(* Logix 5000 Program export KEP; software revision 30.00; part 9 of 15 *)

ADD_ON_INSTRUCTION B256_DINTtoE   (* revision 1.0 20170916, vendor Kenneth A. Fischer *)
// Convert 256-bit value using 8 32-bit pieces into 256-bit value using 32 8-bit pieces
// Revision note:
// Rev1.0: 20170916 - Initial Release
VAR_IN_OUT
   Inp_DINT : DINT[8]; {required}
   Out_E : DINT[32]; {required}
END_VAR
VAR
   i : INT;
   j : INT;
   D_SHR : D_SHR;
   TEMP : DINT;
END_VAR

ROUTINE Logic   (* ladder *)
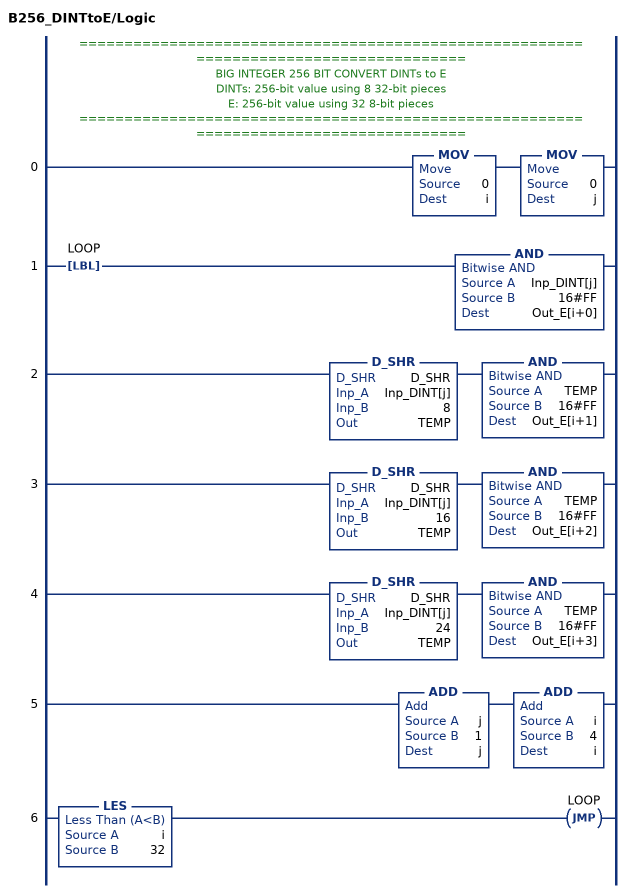
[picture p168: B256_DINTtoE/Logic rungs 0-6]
   // ======================================================================================
   // BIG INTEGER 256 BIT CONVERT DINTs to E
   // DINTs: 256-bit value using 8 32-bit pieces
   // E: 256-bit value using 32 8-bit pieces
   // ======================================================================================
   0: MOV(0,i)MOV(0,j);
   1: LBL(LOOP)AND(Inp_DINT[j],16#FF,Out_E[i+0]);
   2: D_SHR(D_SHR,Inp_DINT[j],8,TEMP)AND(TEMP,16#FF,Out_E[i+1]);
   3: D_SHR(D_SHR,Inp_DINT[j],16,TEMP)AND(TEMP,16#FF,Out_E[i+2]);
   4: D_SHR(D_SHR,Inp_DINT[j],24,TEMP)AND(TEMP,16#FF,Out_E[i+3]);
   5: ADD(j,1,j)ADD(i,4,i);
   6: LES(i,32)JMP(LOOP);
END_ROUTINE
END_ADD_ON_INSTRUCTION

ADD_ON_INSTRUCTION B256_EtoDINT   (* revision 1.0 20170916, vendor Kenneth A. Fischer *)
// Convert 256-bit value using 32 8-bit pieces into 256-bit value using 8 32-bit pieces
// Revision note:
// Rev1.0: 20170916 - Initial Release
VAR_IN_OUT
   Inp_E : DINT[32]; {required}
   Out_DINT : DINT[8]; {required}
END_VAR
VAR
   D_SHL : D_SHL;
   i : INT;
   j : INT;
   TEMP : DINT;
END_VAR

ROUTINE Logic   (* ladder *)
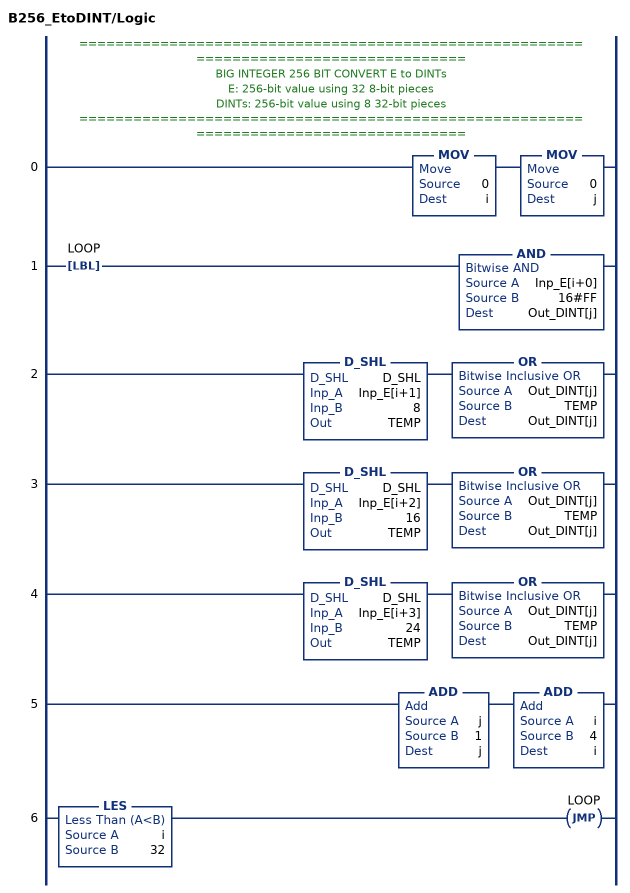
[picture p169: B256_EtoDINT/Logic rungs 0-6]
   // ======================================================================================
   // BIG INTEGER 256 BIT CONVERT E to DINTs
   // E: 256-bit value using 32 8-bit pieces
   // DINTs: 256-bit value using 8 32-bit pieces
   // ======================================================================================
   0: MOV(0,i)MOV(0,j);
   1: LBL(LOOP)AND(Inp_E[i+0],16#FF,Out_DINT[j]);
   2: D_SHL(D_SHL,Inp_E[i+1],8,TEMP)OR(Out_DINT[j],TEMP,Out_DINT[j]);
   3: D_SHL(D_SHL,Inp_E[i+2],16,TEMP)OR(Out_DINT[j],TEMP,Out_DINT[j]);
   4: D_SHL(D_SHL,Inp_E[i+3],24,TEMP)OR(Out_DINT[j],TEMP,Out_DINT[j]);
   5: ADD(j,1,j)ADD(i,4,i);
   6: LES(i,32)JMP(LOOP);
END_ROUTINE
END_ADD_ON_INSTRUCTION

ADD_ON_INSTRUCTION D_ROTR   (* revision 1.0 20170524, vendor Kenneth A. Fischer *)
// DINT circular right shift (rotation) of the 32-bit argument Inp_A by Inp_B bits
// Revision note:
// Rev1.0: 20170524 - Initial Release
VAR_IN_OUT
   Inp_A : DINT; {required}   // 64-bit Integer to be right circular rotated
END_VAR
VAR_INPUT
   Inp_B : INT; {required}   // Number of Inp_A bit rotations
END_VAR
VAR_IN_OUT
   Out : DINT; {required}   // Result
END_VAR
VAR
   Wrk_InpA : DINT[2];
   BSR_Cntrl : CONTROL := (LEN := 32);
   Source_Bit : BOOL;
   ONS : BOOL;
END_VAR

ROUTINE Logic   (* ladder *)
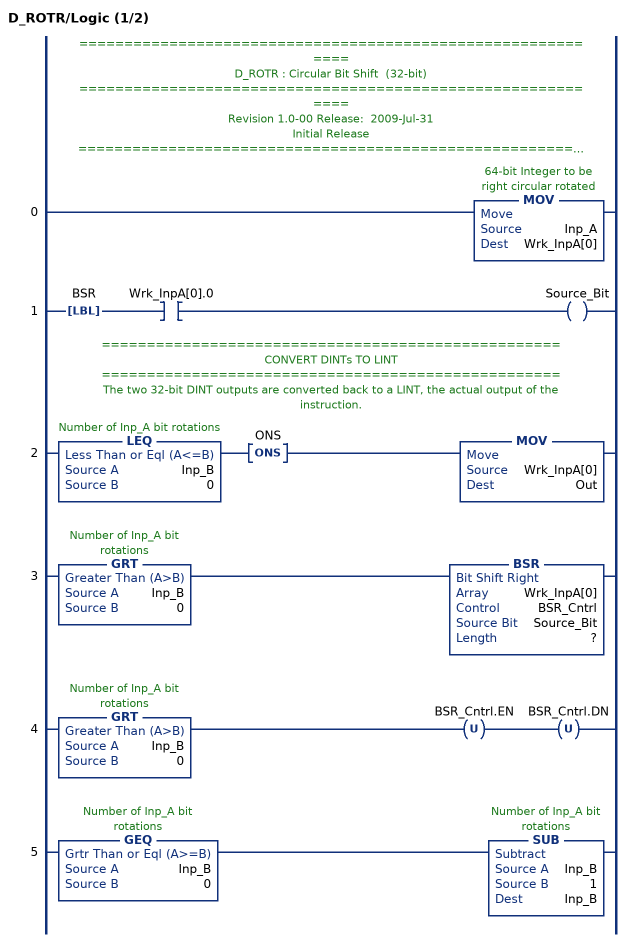
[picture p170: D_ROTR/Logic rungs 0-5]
   // ============================================================
   // D_ROTR : Circular Bit Shift  (32-bit)
   // ============================================================
   // Revision 1.0-00 Release:  2009-Jul-31
   // Initial Release
   // ============================================================
   // Performs a circular right shift rotation of the 32-bit argument Inp_A by the
   // number of bits defined in the 16-bit argument Inp_B.
   0: MOV(Inp_A,Wrk_InpA[0]);
   1: LBL(BSR)XIC(Wrk_InpA[0].0)OTE(Source_Bit);
   // ===================================================
   // CONVERT DINTs TO LINT
   // ===================================================
   // The two 32-bit DINT outputs are converted back to a LINT, the actual output of the instruction.
   2: LEQ(Inp_B,0)ONS(ONS)MOV(Wrk_InpA[0],Out);
   3: GRT(Inp_B,0)BSR(Wrk_InpA[0],BSR_Cntrl,Source_Bit,?);
   4: GRT(Inp_B,0)OTU(BSR_Cntrl.EN)OTU(BSR_Cntrl.DN);
   5: GEQ(Inp_B,0)SUB(Inp_B,1,Inp_B);
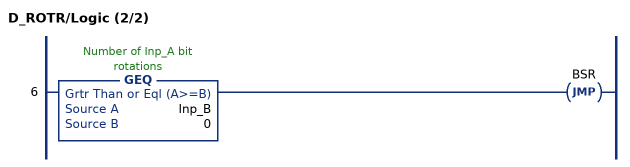
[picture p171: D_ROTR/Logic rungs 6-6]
   6: GEQ(Inp_B,0)JMP(BSR);
END_ROUTINE
END_ADD_ON_INSTRUCTION

ADD_ON_INSTRUCTION VMAC   (* revision 1.0 20170524, vendor Kenneth A. Fischer *)
// Variable Round MAC
// Revision note:
// Rev1.0: 20170524 - Initial Release
VAR_IN_OUT
   Inp_KEY : DINT[8]; {required}
   Inp_MSG : DINT[500]; {required}
END_VAR
VAR_INPUT
   Inp_LEN : DINT; {required}   // LENGTH INPUT OF MSG IN NUMBER OF DINTS
   Inp_ROUNDS : DINT; {required}
END_VAR
VAR_IN_OUT
   Out_VMAC : DINT[8]; {required}
        [0]   // HashBuffer_A
        [1]   // HashBuffer_B
        [2]   // HashBuffer_C
        [3]   // HashBuffer_D
        [4]   // HashBuffer_E
        [5]   // HashBuffer_F
        [6]   // HashBuffer_G
        [7]   // HashBuffer_H
END_VAR
VAR
   MajFunc : DINT;
   HashBuffer_H : DINT;
   HashBuffer_G : DINT;
   HashBuffer_F : DINT;
   HashBuffer_E : DINT;
   HashBuffer_D : DINT;
   HashBuffer_C : DINT;
   HashBuffer_B : DINT;
   HashBuffer_A : DINT;
   W : DINT[64];   // MESSAGE SCHEDULE
   tmp : DINT[20];
   T2 : DINT;
   T1 : DINT;
   t : INT;
   M : INT;   // MESSAGE INCREMENTS
   SigmaE : DINT;
   SigmaA : DINT;
   Sigma1 : DINT;
   Sigma0 : DINT;
   i : INT;
   x : INT;
   HashBufferInput_H : DINT;
   HashBufferInput_G : DINT;
   HashBufferInput_F : DINT;
   HashBufferInput_E : DINT;
   HashBufferInput_D : DINT;
   HashBufferInput_C : DINT;
   HashBufferInput_B : DINT;
   HashBufferInput_A : DINT;
   CondFunc : DINT;
   K : DINT[64];
   LENGTH_BITS : DINT;   // LENGTH OF MSG IN BITS
   LENGTH_MODULO : DINT;
   NUM_PADDING_BITS : DINT;   // NUMBER OF BITS NEEDED FOR PADDING
   NUM_PADDING_DINTS : DINT;   // NUMBER OF DINTS NEEDED FOR PADDING
   PADDING_COUNTER : DINT;
   TOTAL_MSG_LENGTH_MINUS_16 : DINT;
   D_ROTR : D_ROTR;
   D_SHR : D_SHR;
   ROUNDS : DINT;
   n : INT;
   KeyIndex : DINT;
   RotationIndex : DINT;
   IndexedKey : DINT;
END_VAR

ROUTINE Logic   (* ladder *)
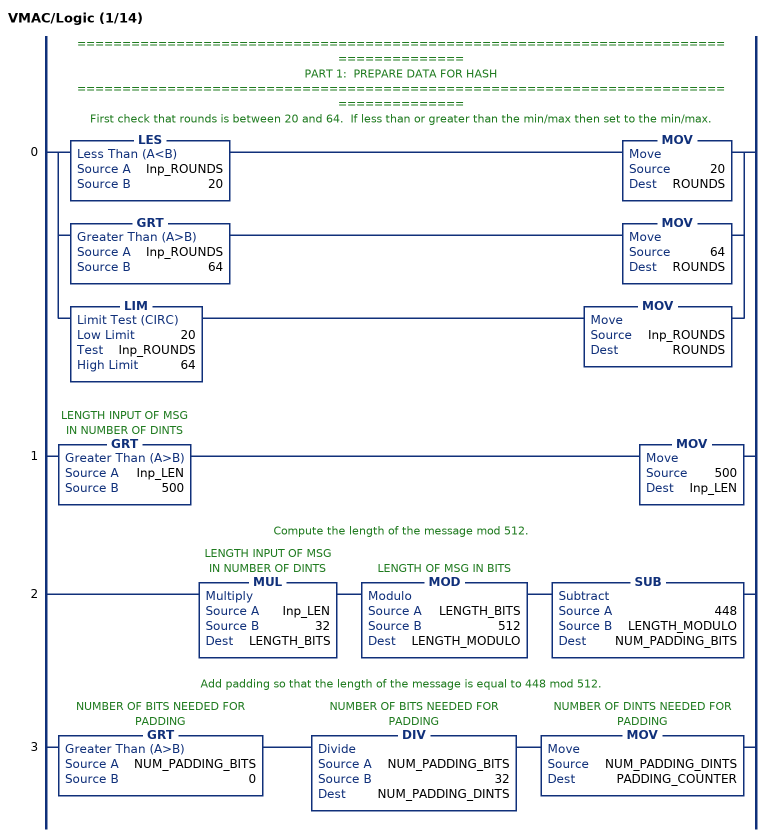
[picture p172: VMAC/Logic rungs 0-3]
   // ======================================================================================
   // PART 1:  PREPARE DATA FOR HASH
   // ======================================================================================
   // First check that rounds is between 20 and 64.  If less than or greater than the min/max then set to the min/max.
   0: [LES(Inp_ROUNDS,20) MOV(20,ROUNDS) ,GRT(Inp_ROUNDS,64) MOV(64,ROUNDS) ,LIM(20,Inp_ROUNDS,64) MOV(Inp_ROUNDS,ROUNDS) ];
   1: GRT(Inp_LEN,500)MOV(500,Inp_LEN);
   // Compute the length of the message mod 512.
   2: MUL(Inp_LEN,32,LENGTH_BITS)MOD(LENGTH_BITS,512,LENGTH_MODULO)SUB(448,LENGTH_MODULO,NUM_PADDING_BITS);
   // Add padding so that the length of the message is equal to 448 mod 512.
   3: GRT(NUM_PADDING_BITS,0)DIV(NUM_PADDING_BITS,32,NUM_PADDING_DINTS)MOV(NUM_PADDING_DINTS,PADDING_COUNTER);
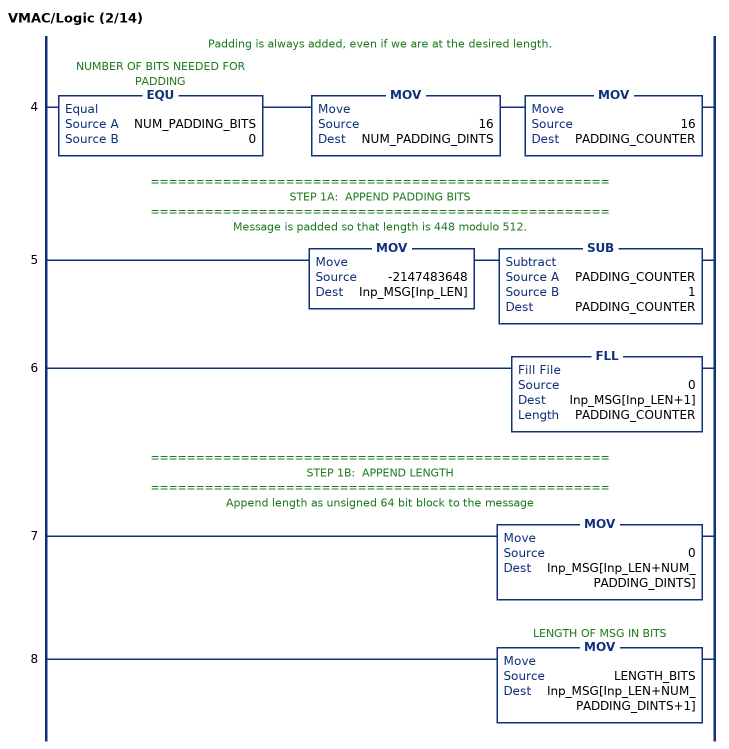
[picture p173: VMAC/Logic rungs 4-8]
   // Padding is always added, even if we are at the desired length.
   4: EQU(NUM_PADDING_BITS,0)MOV(16,NUM_PADDING_DINTS)MOV(16,PADDING_COUNTER);
   // ===================================================
   // STEP 1A:  APPEND PADDING BITS
   // ===================================================
   // Message is padded so that length is 448 modulo 512.
   5: MOV(-2147483648,Inp_MSG[Inp_LEN])SUB(PADDING_COUNTER,1,PADDING_COUNTER);
   6: FLL(0,Inp_MSG[Inp_LEN+1],PADDING_COUNTER);
   // ===================================================
   // STEP 1B:  APPEND LENGTH
   // ===================================================
   // Append length as unsigned 64 bit block to the message
   7: MOV(0,Inp_MSG[Inp_LEN+NUM_PADDING_DINTS]);
   8: MOV(LENGTH_BITS,Inp_MSG[Inp_LEN+NUM_PADDING_DINTS+1]);
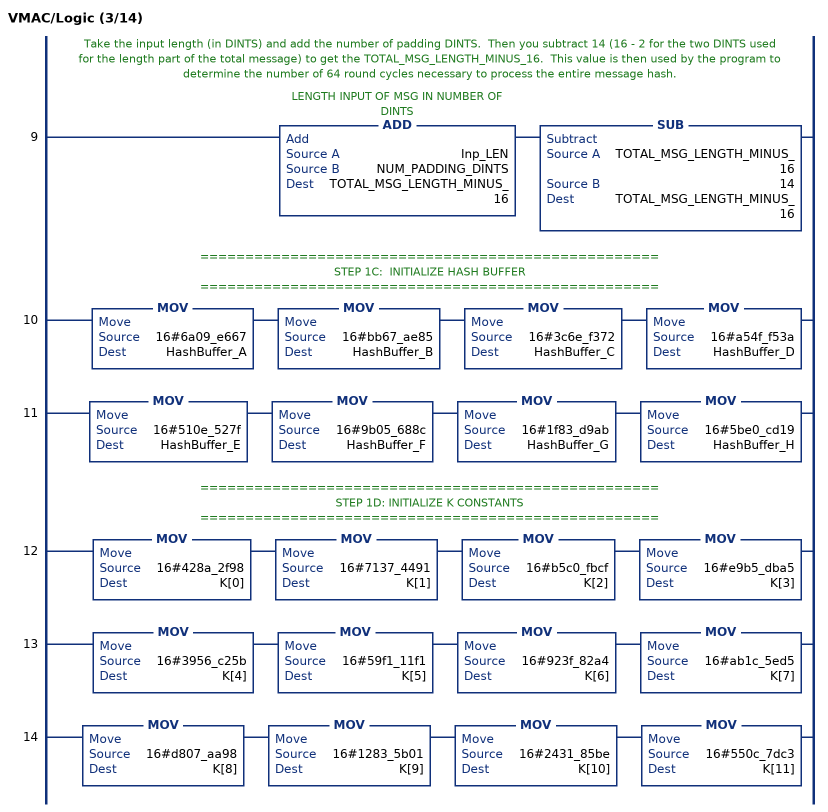
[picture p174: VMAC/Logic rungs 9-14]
   // Take the input length (in DINTS) and add the number of padding DINTS.  Then you subtract 14 (16 - 2 for the two DINTS used for the length part of the total message) to get the TOTAL_MSG_LENGTH_MINUS_16.  This value is then used by the program to determine the number of 64 round cycles necessary to process the entire message hash.
   9: ADD(Inp_LEN,NUM_PADDING_DINTS,TOTAL_MSG_LENGTH_MINUS_16)SUB(TOTAL_MSG_LENGTH_MINUS_16,14,TOTAL_MSG_LENGTH_MINUS_16);
   // ===================================================
   // STEP 1C:  INITIALIZE HASH BUFFER
   // ===================================================
   10: MOV(16#6a09_e667,HashBuffer_A)MOV(16#bb67_ae85,HashBuffer_B)MOV(16#3c6e_f372,HashBuffer_C)MOV(16#a54f_f53a,HashBuffer_D);
   11: MOV(16#510e_527f,HashBuffer_E)MOV(16#9b05_688c,HashBuffer_F)MOV(16#1f83_d9ab,HashBuffer_G)MOV(16#5be0_cd19,HashBuffer_H);
   // ===================================================
   // STEP 1D: INITIALIZE K CONSTANTS
   // ===================================================
   12: MOV(16#428a_2f98,K[0])MOV(16#7137_4491,K[1])MOV(16#b5c0_fbcf,K[2])MOV(16#e9b5_dba5,K[3]);
   13: MOV(16#3956_c25b,K[4])MOV(16#59f1_11f1,K[5])MOV(16#923f_82a4,K[6])MOV(16#ab1c_5ed5,K[7]);
   14: MOV(16#d807_aa98,K[8])MOV(16#1283_5b01,K[9])MOV(16#2431_85be,K[10])MOV(16#550c_7dc3,K[11]);
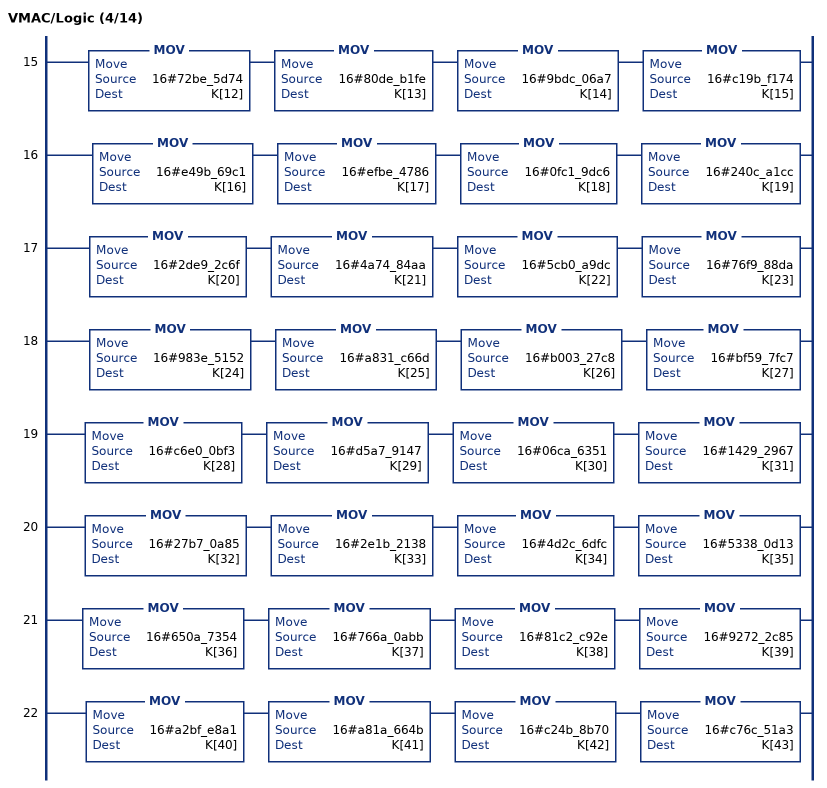
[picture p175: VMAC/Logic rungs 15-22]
   15: MOV(16#72be_5d74,K[12])MOV(16#80de_b1fe,K[13])MOV(16#9bdc_06a7,K[14])MOV(16#c19b_f174,K[15]);
   16: MOV(16#e49b_69c1,K[16])MOV(16#efbe_4786,K[17])MOV(16#0fc1_9dc6,K[18])MOV(16#240c_a1cc,K[19]);
   17: MOV(16#2de9_2c6f,K[20])MOV(16#4a74_84aa,K[21])MOV(16#5cb0_a9dc,K[22])MOV(16#76f9_88da,K[23]);
   18: MOV(16#983e_5152,K[24])MOV(16#a831_c66d,K[25])MOV(16#b003_27c8,K[26])MOV(16#bf59_7fc7,K[27]);
   19: MOV(16#c6e0_0bf3,K[28])MOV(16#d5a7_9147,K[29])MOV(16#06ca_6351,K[30])MOV(16#1429_2967,K[31]);
   20: MOV(16#27b7_0a85,K[32])MOV(16#2e1b_2138,K[33])MOV(16#4d2c_6dfc,K[34])MOV(16#5338_0d13,K[35]);
   21: MOV(16#650a_7354,K[36])MOV(16#766a_0abb,K[37])MOV(16#81c2_c92e,K[38])MOV(16#9272_2c85,K[39]);
   22: MOV(16#a2bf_e8a1,K[40])MOV(16#a81a_664b,K[41])MOV(16#c24b_8b70,K[42])MOV(16#c76c_51a3,K[43]);
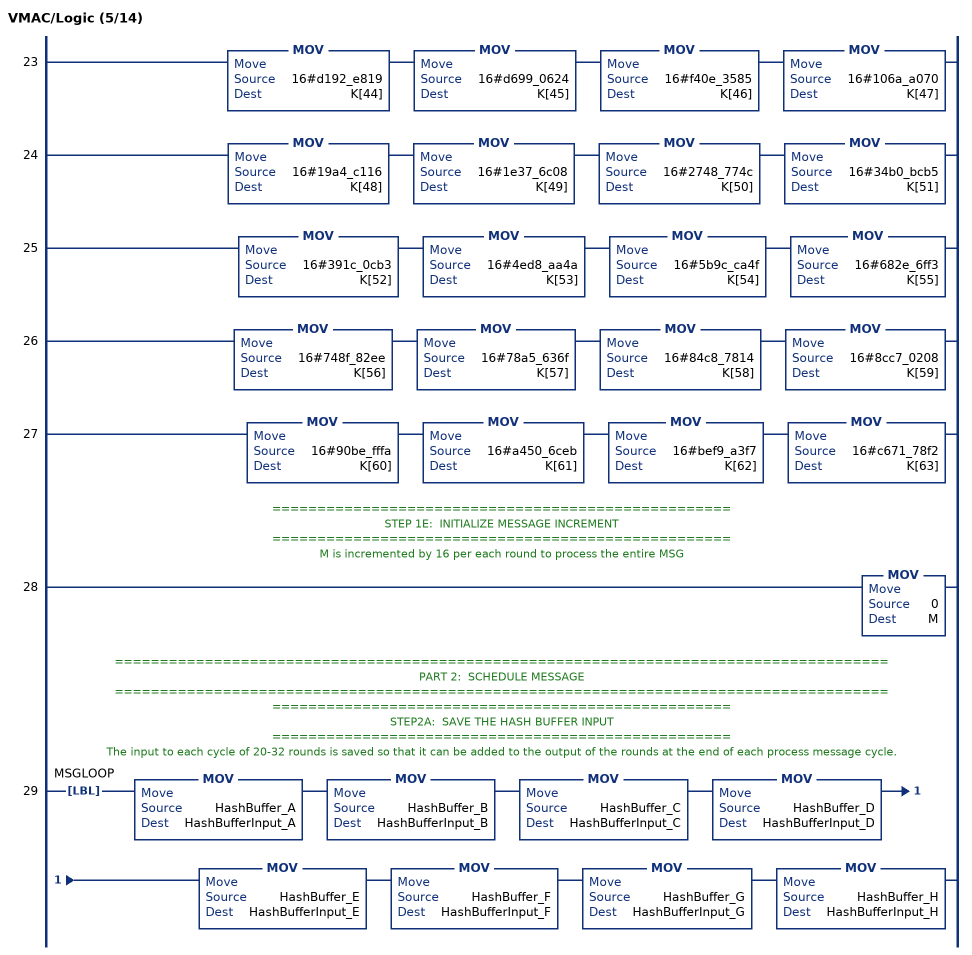
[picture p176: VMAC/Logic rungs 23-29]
   23: MOV(16#d192_e819,K[44])MOV(16#d699_0624,K[45])MOV(16#f40e_3585,K[46])MOV(16#106a_a070,K[47]);
   24: MOV(16#19a4_c116,K[48])MOV(16#1e37_6c08,K[49])MOV(16#2748_774c,K[50])MOV(16#34b0_bcb5,K[51]);
   25: MOV(16#391c_0cb3,K[52])MOV(16#4ed8_aa4a,K[53])MOV(16#5b9c_ca4f,K[54])MOV(16#682e_6ff3,K[55]);
   26: MOV(16#748f_82ee,K[56])MOV(16#78a5_636f,K[57])MOV(16#84c8_7814,K[58])MOV(16#8cc7_0208,K[59]);
   27: MOV(16#90be_fffa,K[60])MOV(16#a450_6ceb,K[61])MOV(16#bef9_a3f7,K[62])MOV(16#c671_78f2,K[63]);
   // ===================================================
   // STEP 1E:  INITIALIZE MESSAGE INCREMENT
   // ===================================================
   // M is incremented by 16 per each round to process the entire MSG
   28: MOV(0,M);
   // ======================================================================================
   // PART 2:  SCHEDULE MESSAGE
   // ======================================================================================
   // ===================================================
   // STEP2A:  SAVE THE HASH BUFFER INPUT
   // ===================================================
   // The input to each cycle of 20-32 rounds is saved so that it can be added to the output of the rounds at the end of each process message cycle.
   29: LBL(MSGLOOP)MOV(HashBuffer_A,HashBufferInput_A)MOV(HashBuffer_B,HashBufferInput_B)MOV(HashBuffer_C,HashBufferInput_C)MOV(HashBuffer_D,HashBufferInput_D)MOV(HashBuffer_E,HashBufferInput_E)MOV(HashBuffer_F,HashBufferInput_F)MOV(HashBuffer_G,HashBufferInput_G)MOV(HashBuffer_H,HashBufferInput_H);
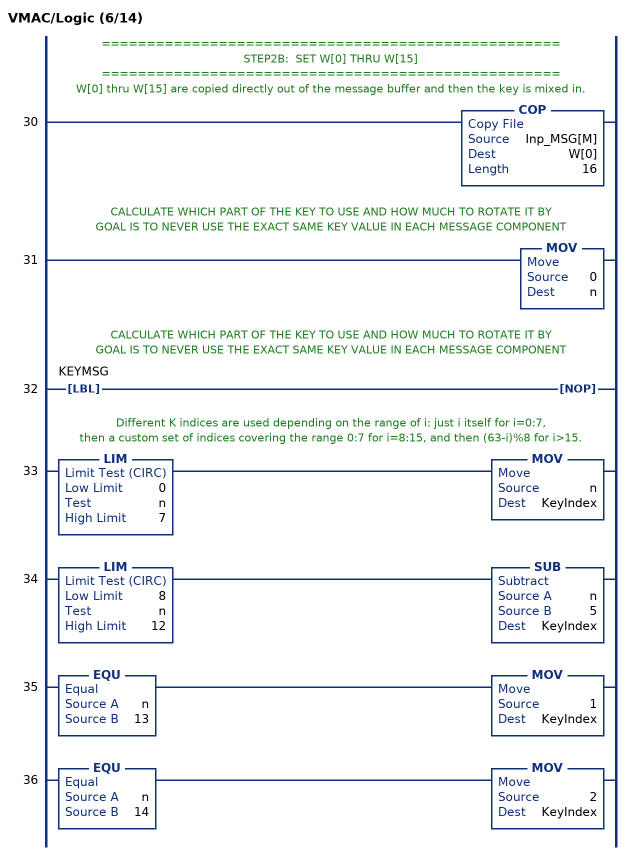
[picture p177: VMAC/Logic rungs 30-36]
   // ===================================================
   // STEP2B:  SET W[0] THRU W[15]
   // ===================================================
   // W[0] thru W[15] are copied directly out of the message buffer and then the key is mixed in.
   30: COP(Inp_MSG[M],W[0],16);
   // CALCULATE WHICH PART OF THE KEY TO USE AND HOW MUCH TO ROTATE IT BY
   // GOAL IS TO NEVER USE THE EXACT SAME KEY VALUE IN EACH MESSAGE COMPONENT
   31: MOV(0,n);
   // CALCULATE WHICH PART OF THE KEY TO USE AND HOW MUCH TO ROTATE IT BY
   // GOAL IS TO NEVER USE THE EXACT SAME KEY VALUE IN EACH MESSAGE COMPONENT
   32: LBL(KEYMSG)NOP();
   // Different K indices are used depending on the range of i: just i itself for i=0:7,
   // then a custom set of indices covering the range 0:7 for i=8:15, and then (63-i)%8 for i>15.
   33: LIM(0,n,7)MOV(n,KeyIndex);
   34: LIM(8,n,12)SUB(n,5,KeyIndex);
   35: EQU(n,13)MOV(1,KeyIndex);
   36: EQU(n,14)MOV(2,KeyIndex);
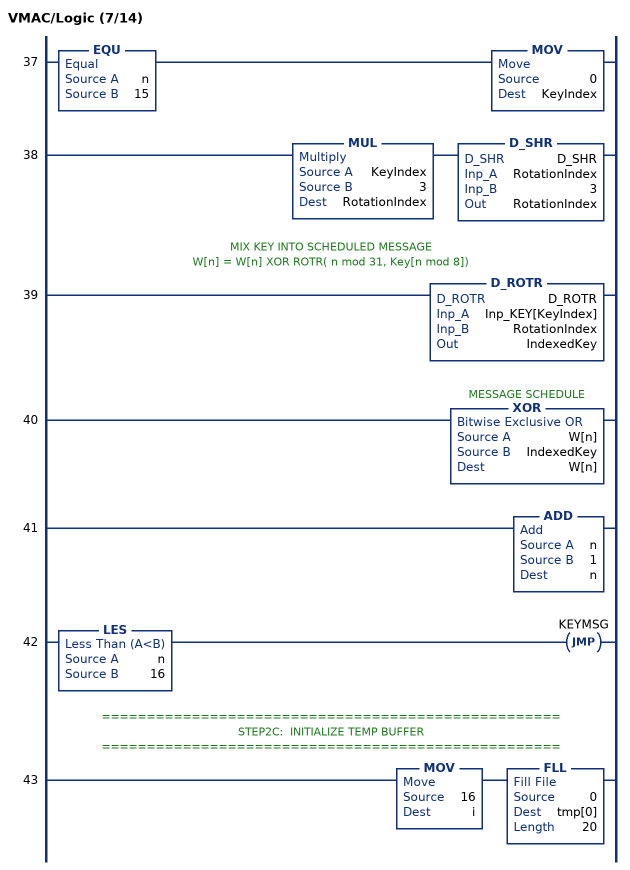
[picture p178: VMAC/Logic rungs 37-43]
   37: EQU(n,15)MOV(0,KeyIndex);
   38: MUL(KeyIndex,3,RotationIndex)D_SHR(D_SHR,RotationIndex,3,RotationIndex);
   // MIX KEY INTO SCHEDULED MESSAGE
   // W[n] = W[n] XOR ROTR( n mod 31, Key[n mod 8])
   39: D_ROTR(D_ROTR,Inp_KEY[KeyIndex],RotationIndex,IndexedKey);
   40: XOR(W[n],IndexedKey,W[n]);
   41: ADD(n,1,n);
   42: LES(n,16)JMP(KEYMSG);
   // ===================================================
   // STEP2C:  INITIALIZE TEMP BUFFER
   // ===================================================
   43: MOV(16,i)FLL(0,tmp[0],20);
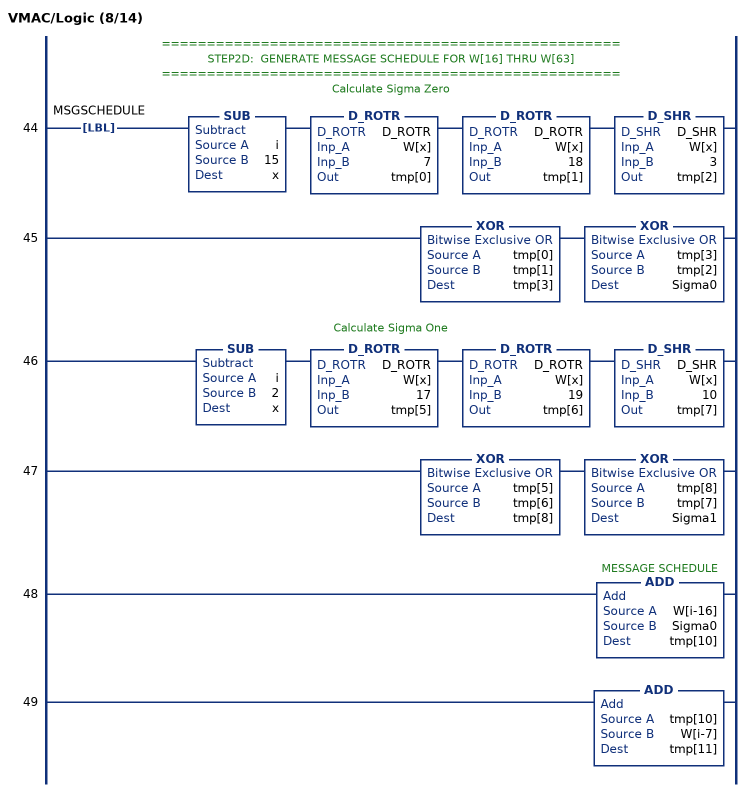
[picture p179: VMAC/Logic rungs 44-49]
   // ===================================================
   // STEP2D:  GENERATE MESSAGE SCHEDULE FOR W[16] THRU W[63]
   // ===================================================
   // Calculate Sigma Zero
   44: LBL(MSGSCHEDULE)SUB(i,15,x)D_ROTR(D_ROTR,W[x],7,tmp[0])D_ROTR(D_ROTR,W[x],18,tmp[1])D_SHR(D_SHR,W[x],3,tmp[2]);
   45: XOR(tmp[0],tmp[1],tmp[3])XOR(tmp[3],tmp[2],Sigma0);
   // Calculate Sigma One
   46: SUB(i,2,x)D_ROTR(D_ROTR,W[x],17,tmp[5])D_ROTR(D_ROTR,W[x],19,tmp[6])D_SHR(D_SHR,W[x],10,tmp[7]);
   47: XOR(tmp[5],tmp[6],tmp[8])XOR(tmp[8],tmp[7],Sigma1);
   48: ADD(W[i-16],Sigma0,tmp[10]);
   49: ADD(tmp[10],W[i-7],tmp[11]);
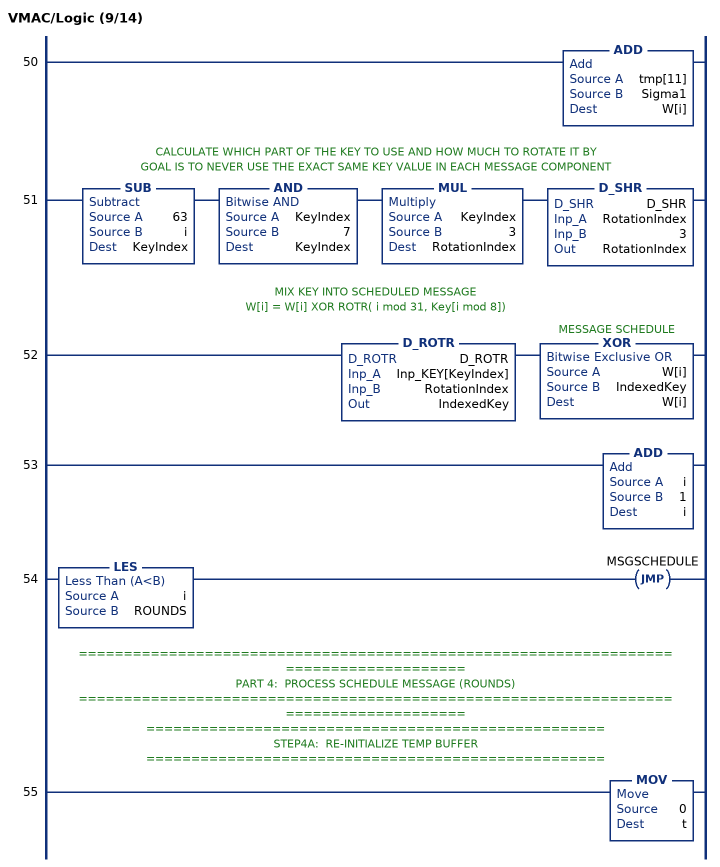
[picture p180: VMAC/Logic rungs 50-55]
   50: ADD(tmp[11],Sigma1,W[i]);
   // CALCULATE WHICH PART OF THE KEY TO USE AND HOW MUCH TO ROTATE IT BY
   // GOAL IS TO NEVER USE THE EXACT SAME KEY VALUE IN EACH MESSAGE COMPONENT
   51: SUB(63,i,KeyIndex)AND(KeyIndex,7,KeyIndex)MUL(KeyIndex,3,RotationIndex)D_SHR(D_SHR,RotationIndex,3,RotationIndex);
   // MIX KEY INTO SCHEDULED MESSAGE
   // W[i] = W[i] XOR ROTR( i mod 31, Key[i mod 8])
   52: D_ROTR(D_ROTR,Inp_KEY[KeyIndex],RotationIndex,IndexedKey)XOR(W[i],IndexedKey,W[i]);
   53: ADD(i,1,i);
   54: LES(i,ROUNDS)JMP(MSGSCHEDULE);
   // ======================================================================================
   // PART 4:  PROCESS SCHEDULE MESSAGE (ROUNDS)
   // ======================================================================================
   // ===================================================
   // STEP4A:  RE-INITIALIZE TEMP BUFFER
   // ===================================================
   55: MOV(0,t);
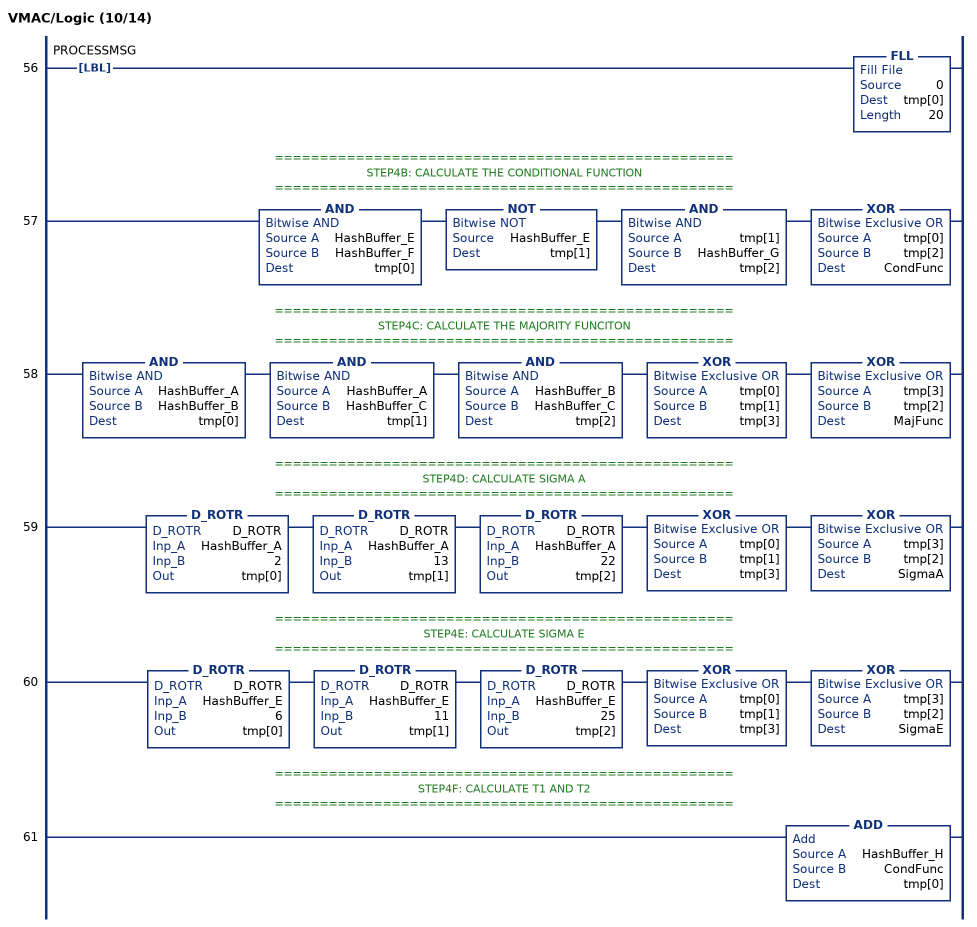
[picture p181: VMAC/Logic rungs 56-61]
   56: LBL(PROCESSMSG)FLL(0,tmp[0],20);
   // ===================================================
   // STEP4B: CALCULATE THE CONDITIONAL FUNCTION
   // ===================================================
   57: AND(HashBuffer_E,HashBuffer_F,tmp[0])NOT(HashBuffer_E,tmp[1])AND(tmp[1],HashBuffer_G,tmp[2])XOR(tmp[0],tmp[2],CondFunc);
   // ===================================================
   // STEP4C: CALCULATE THE MAJORITY FUNCITON
   // ===================================================
   58: AND(HashBuffer_A,HashBuffer_B,tmp[0])AND(HashBuffer_A,HashBuffer_C,tmp[1])AND(HashBuffer_B,HashBuffer_C,tmp[2])XOR(tmp[0],tmp[1],tmp[3])XOR(tmp[3],tmp[2],MajFunc);
   // ===================================================
   // STEP4D: CALCULATE SIGMA A
   // ===================================================
   59: D_ROTR(D_ROTR,HashBuffer_A,2,tmp[0])D_ROTR(D_ROTR,HashBuffer_A,13,tmp[1])D_ROTR(D_ROTR,HashBuffer_A,22,tmp[2])XOR(tmp[0],tmp[1],tmp[3])XOR(tmp[3],tmp[2],SigmaA);
   // ===================================================
   // STEP4E: CALCULATE SIGMA E
   // ===================================================
   60: D_ROTR(D_ROTR,HashBuffer_E,6,tmp[0])D_ROTR(D_ROTR,HashBuffer_E,11,tmp[1])D_ROTR(D_ROTR,HashBuffer_E,25,tmp[2])XOR(tmp[0],tmp[1],tmp[3])XOR(tmp[3],tmp[2],SigmaE);
   // ===================================================
   // STEP4F: CALCULATE T1 AND T2
   // ===================================================
   61: ADD(HashBuffer_H,CondFunc,tmp[0]);
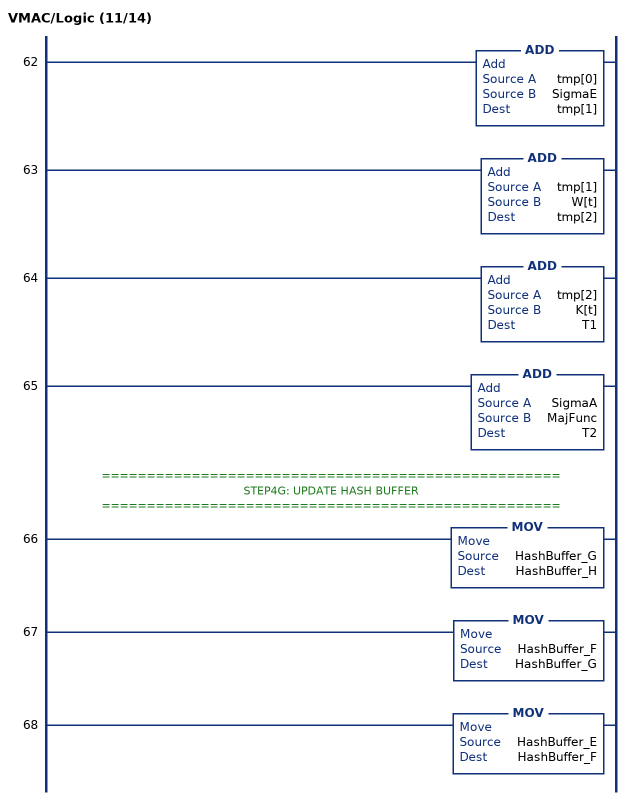
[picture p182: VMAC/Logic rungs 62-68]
   62: ADD(tmp[0],SigmaE,tmp[1]);
   63: ADD(tmp[1],W[t],tmp[2]);
   64: ADD(tmp[2],K[t],T1);
   65: ADD(SigmaA,MajFunc,T2);
   // ===================================================
   // STEP4G: UPDATE HASH BUFFER
   // ===================================================
   66: MOV(HashBuffer_G,HashBuffer_H);
   67: MOV(HashBuffer_F,HashBuffer_G);
   68: MOV(HashBuffer_E,HashBuffer_F);
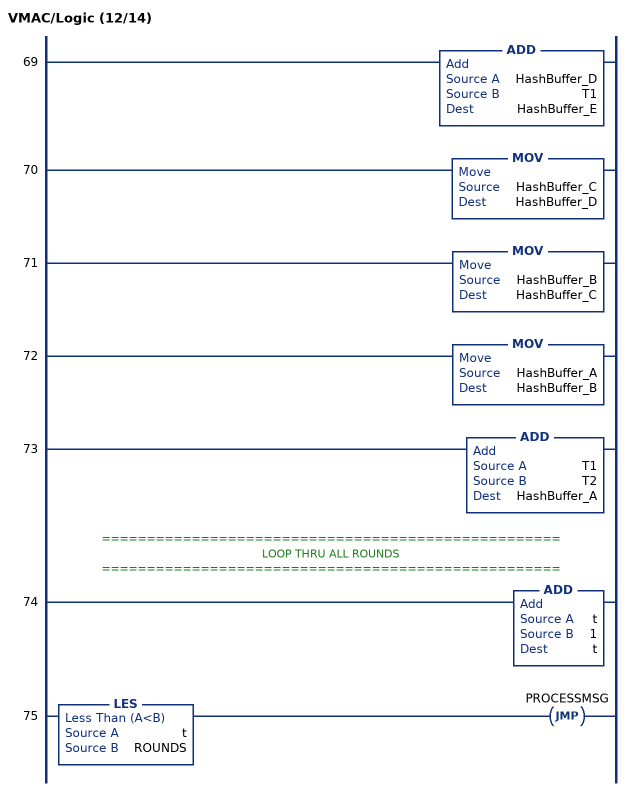
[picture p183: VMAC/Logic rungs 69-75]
   69: ADD(HashBuffer_D,T1,HashBuffer_E);
   70: MOV(HashBuffer_C,HashBuffer_D);
   71: MOV(HashBuffer_B,HashBuffer_C);
   72: MOV(HashBuffer_A,HashBuffer_B);
   73: ADD(T1,T2,HashBuffer_A);
   // ===================================================
   // LOOP THRU ALL ROUNDS
   // ===================================================
   74: ADD(t,1,t);
   75: LES(t,ROUNDS)JMP(PROCESSMSG);
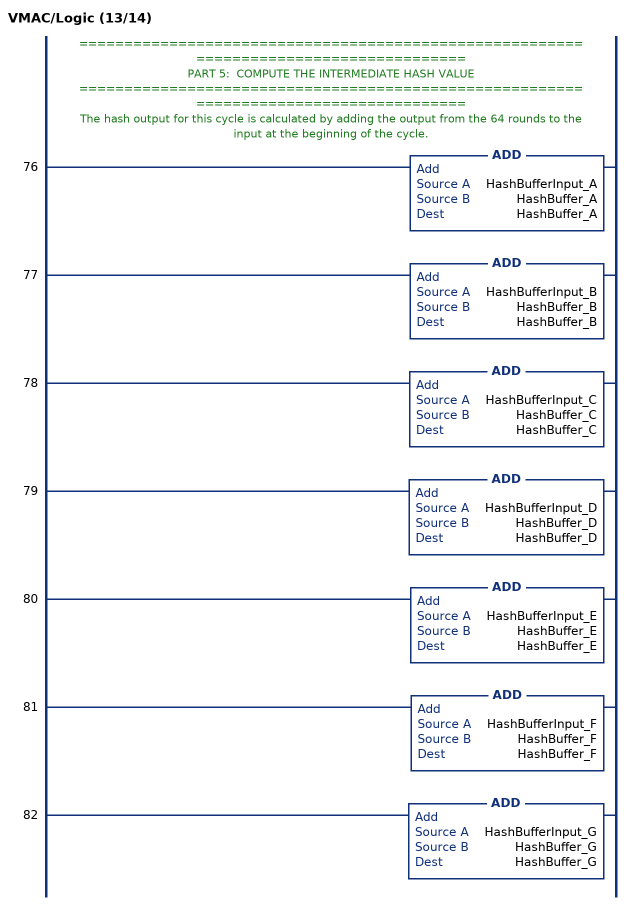
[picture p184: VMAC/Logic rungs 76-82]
   // ======================================================================================
   // PART 5:  COMPUTE THE INTERMEDIATE HASH VALUE
   // ======================================================================================
   // The hash output for this cycle is calculated by adding the output from the 64 rounds to the input at the beginning of the cycle.
   76: ADD(HashBufferInput_A,HashBuffer_A,HashBuffer_A);
   77: ADD(HashBufferInput_B,HashBuffer_B,HashBuffer_B);
   78: ADD(HashBufferInput_C,HashBuffer_C,HashBuffer_C);
   79: ADD(HashBufferInput_D,HashBuffer_D,HashBuffer_D);
   80: ADD(HashBufferInput_E,HashBuffer_E,HashBuffer_E);
   81: ADD(HashBufferInput_F,HashBuffer_F,HashBuffer_F);
   82: ADD(HashBufferInput_G,HashBuffer_G,HashBuffer_G);
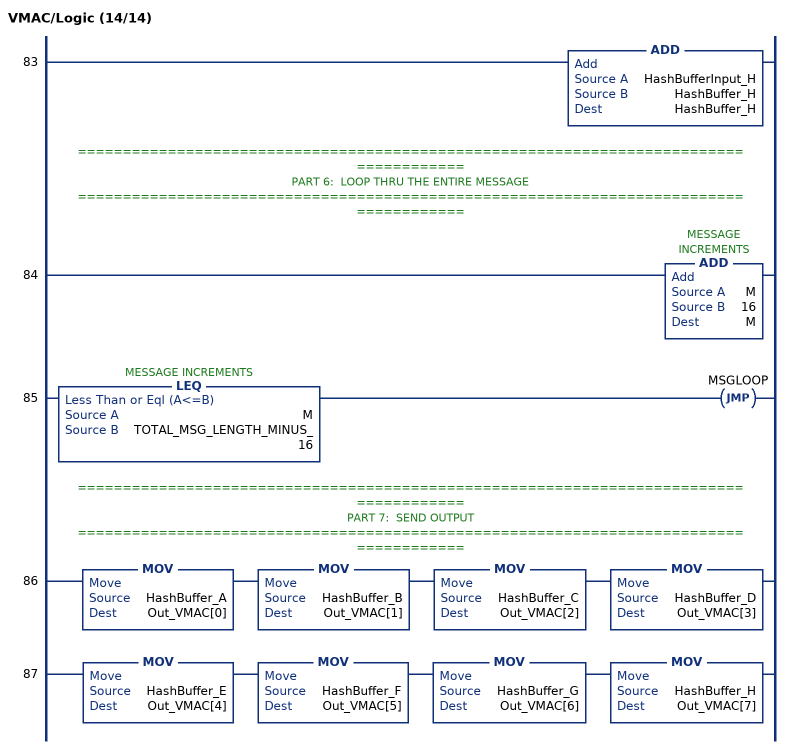
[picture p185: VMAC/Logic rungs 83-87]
   83: ADD(HashBufferInput_H,HashBuffer_H,HashBuffer_H);
   // ======================================================================================
   // PART 6:  LOOP THRU THE ENTIRE MESSAGE
   // ======================================================================================
   84: ADD(M,16,M);
   85: LEQ(M,TOTAL_MSG_LENGTH_MINUS_16)JMP(MSGLOOP);
   // ======================================================================================
   // PART 7:  SEND OUTPUT
   // ======================================================================================
   86: MOV(HashBuffer_A,Out_VMAC[0])MOV(HashBuffer_B,Out_VMAC[1])MOV(HashBuffer_C,Out_VMAC[2])MOV(HashBuffer_D,Out_VMAC[3]);
   87: MOV(HashBuffer_E,Out_VMAC[4])MOV(HashBuffer_F,Out_VMAC[5])MOV(HashBuffer_G,Out_VMAC[6])MOV(HashBuffer_H,Out_VMAC[7]);
END_ROUTINE
END_ADD_ON_INSTRUCTION
